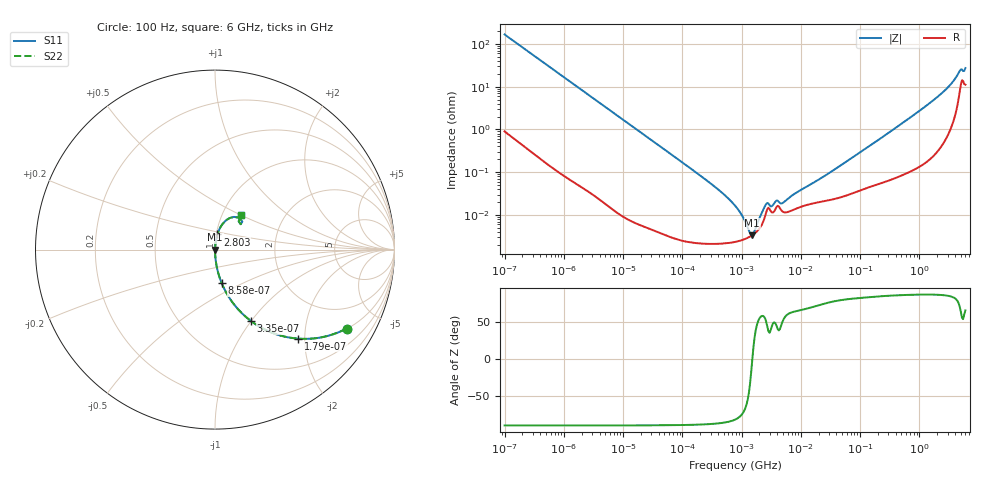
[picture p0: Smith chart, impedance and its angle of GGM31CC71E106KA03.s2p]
!Murata Part Number: GGM31CC71E106KA03
!These Parameters are Measured in Series Mode Connection
!Data Generated on Mar 13, 2026
!  o--ll--o
!Port1  Port2
!  o------o
!Operation Temp=25[degC], DC Bias Voltage=0[V]
!Freq. Start=100[Hz] Stop=6[GHz] 401[Steps]
# Hz S RI R 50
!Freq.(Hz) S11(Real) S11(Imag) S21(Real) S21(Imag) S12(Real) S12(Imag) S22(Real) S22(Imag)
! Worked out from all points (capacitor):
!   401 points, 100 Hz to 6 GHz, reference 50 ohm
!   read as one part in series: C = 9.56 uF near 109 Hz
!   lowest |Z| = 3.36 mohm at 1.516 MHz (marker M1)
!   series resonance near 1.519 MHz, so ESL is about 1.1 nH
!   S11 on the Smith chart (normalised r, x): 100 Hz: 1.02, -3.32; 179 Hz: 1.01, -1.86; 335 Hz: 1.00, -1.00; 858 Hz: 1.00, -0.39; 2.803 GHz: 1.01, +0.17; 6 GHz: 1.22, +0.50
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100  0.7331 -0.4396  0.2669 0.4396  0.2669 0.4396  0.7331 -0.4396
179  0.4641 -0.4961  0.5359 0.4961  0.5359 0.4961  0.4641 -0.4961
335  0.2 -0.3975  0.8 0.3975  0.8 0.3975  0.2 -0.3975
858  0.0375 -0.1875  0.9625 0.1875  0.9625 0.1875  0.0375 -0.1875
2008  0.00736 -0.0829  0.9926 0.0829  0.9926 0.0829  0.00736 -0.0829
40335  5.62e-05 -0.00419  0.9999 0.00419  0.9999 0.00419  5.62e-05 -0.00419
330837  2.12e-05 -0.00049  1 0.00049  1 0.00049  2.12e-05 -0.00049
774597  2.33e-05 -0.000164  1 0.000164  1 0.000164  2.33e-05 -0.000164
1059725  2.63e-05 -8.36e-05  1 8.36e-05  1 8.36e-05  2.63e-05 -8.36e-05
1516199  3.36e-05 -4e-07  1 4e-07  1 4e-07  3.36e-05 -4e-07
2074311  5.16e-05 7.85e-05  0.9999 -7.85e-05  0.9999 -7.85e-05  5.16e-05 7.85e-05
2713602  0.000136 0.000133  0.9999 -0.000133  0.9999 -0.000133  0.000136 0.000133
3245845  0.000114 0.000112  0.9999 -0.000112  0.9999 -0.000112  0.000114 0.000112
3882480  0.000152 0.000153  0.9998 -0.000153  0.9998 -0.000153  0.000152 0.000153
5079039  0.000117 0.000156  0.9999 -0.000156  0.9999 -0.000156  0.000117 0.000156
1.555665e7  0.000184 0.000512  0.9998 -0.000512  0.9998 -0.000512  0.000184 0.000512
3.124326e8  0.000716 0.00854  0.9993 -0.00854  0.9993 -0.00854  0.000716 0.00854
1.309207e9  0.00296 0.0355  0.997 -0.0355  0.997 -0.0355  0.00296 0.0355
2.802721e9  0.0131 0.0842  0.9869 -0.0842  0.9869 -0.0842  0.0131 0.0842
4.009986e9  0.0415 0.1418  0.9585 -0.1418  0.9585 -0.1418  0.0415 0.1418
4.796499e9  0.1059 0.1825  0.8941 -0.1825  0.8941 -0.1825  0.1059 0.1825
6e9  0.143 0.1915  0.857 -0.1915  0.857 -0.1915  0.143 0.1915
